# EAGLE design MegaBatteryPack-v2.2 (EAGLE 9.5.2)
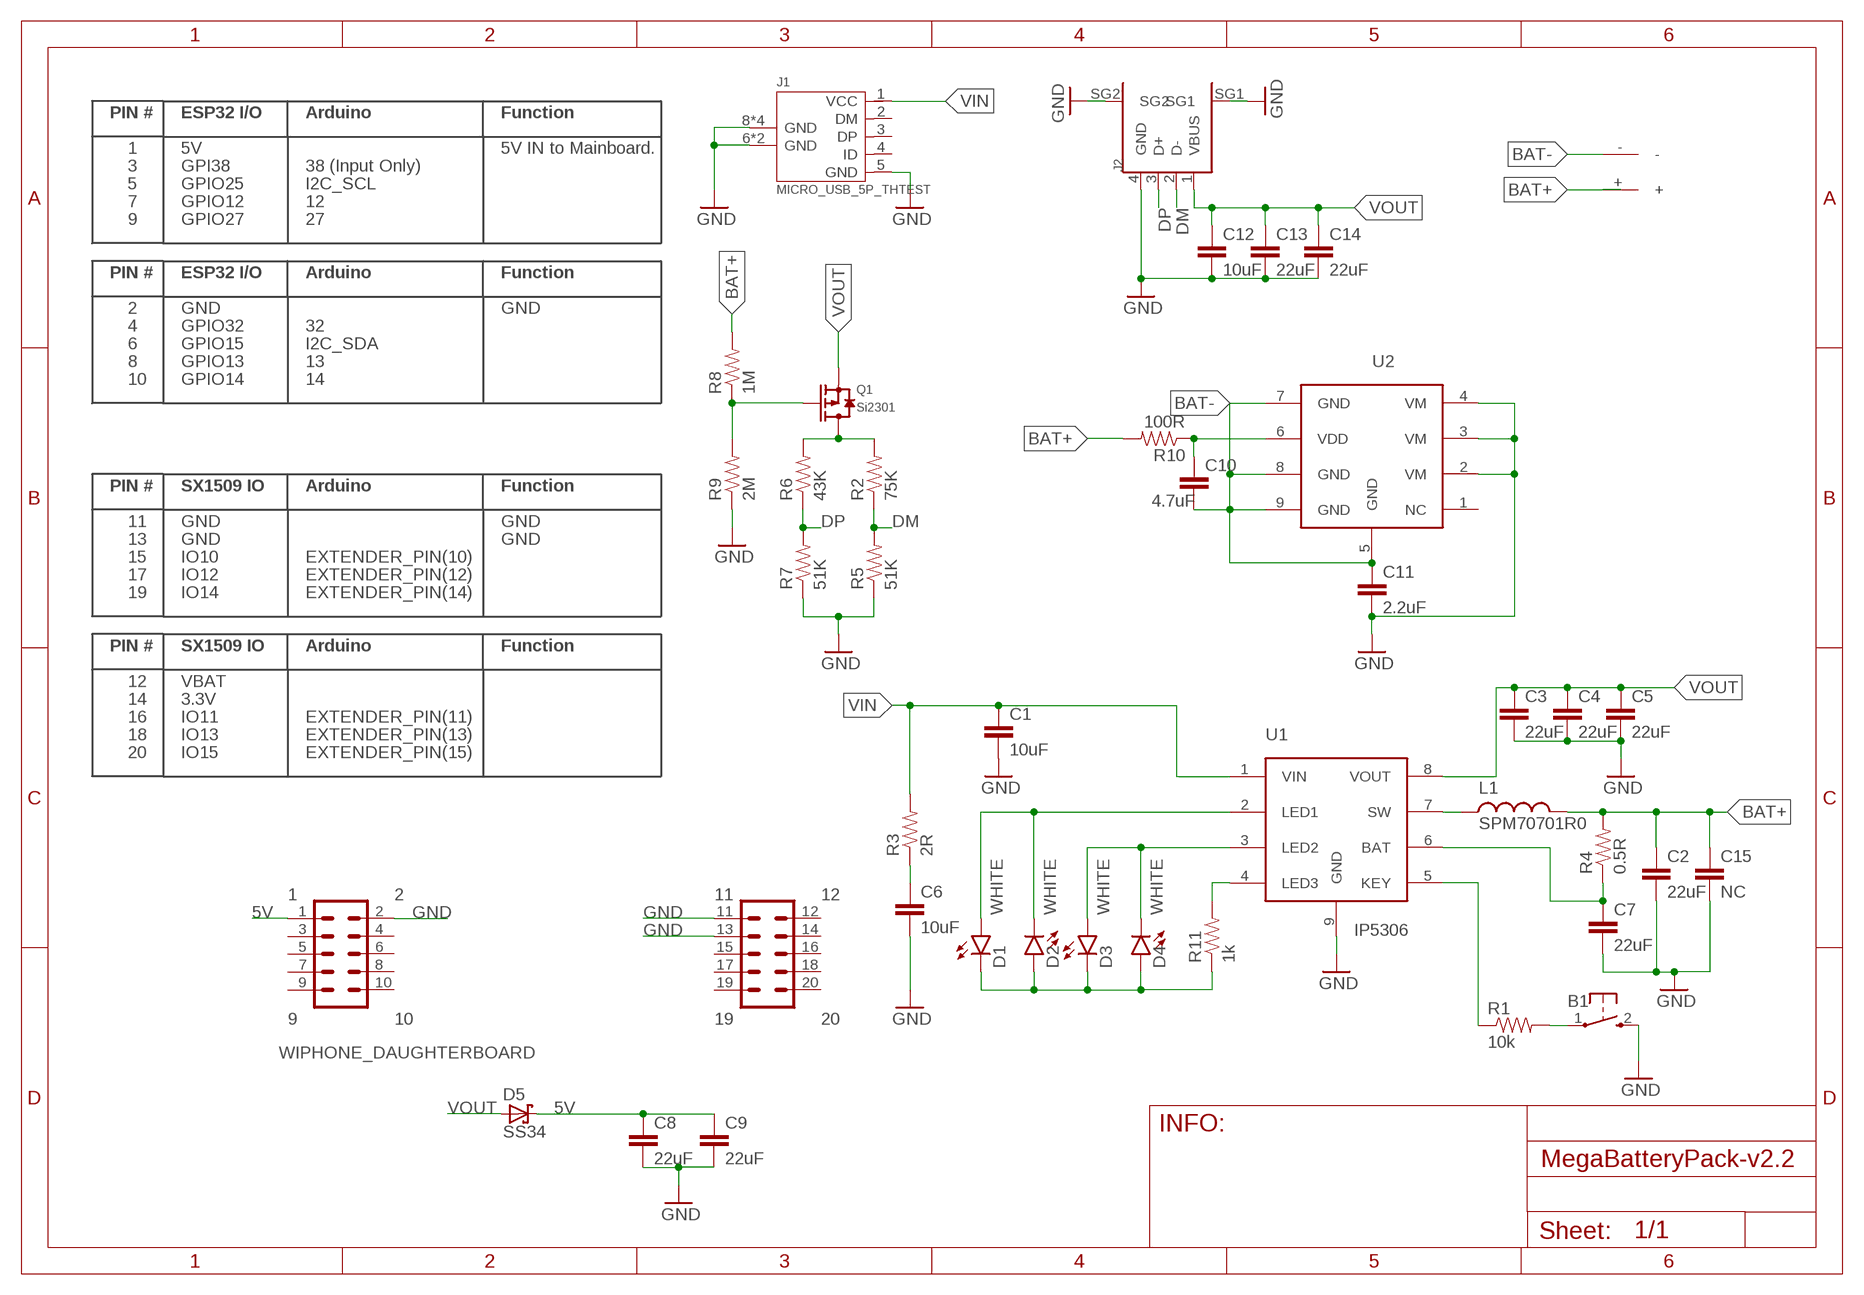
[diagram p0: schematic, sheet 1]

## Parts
B1  BUTTON_3X6X5-90_DEGREE  [3X6X5-90_DEGREE]
C1  10uF  CAP0805  [0805_CAP]
C2  22uF  CAP0805  [0805_CAP]
C3  22uF  CAP0805  [0805_CAP]
C4  22uF  CAP0805  [0805_CAP]
C5  22uF  CAP0805  [0805_CAP]
C6  10uF  CAP0805  [0805_CAP]
C7  22uF  CAP0805  [0805_CAP]
C8  22uF  CAP0805  [0805_CAP]
C9  22uF  CAP0805  [0805_CAP]
C10  4.7uF  CAP  [0603-CAP-L]
C11  2.2uF  CAP0805  [0805_CAP]
C12  10uF  CAP0805  [0805_CAP]
C13  22uF  CAP0805  [0805_CAP]
C14  22uF  CAP0805  [0805_CAP]
C15  NC  CAP0805  [0805_CAP]
D1  WHITE  LED-WHITE0603  [LED-0603]
D2  WHITE  LED-WHITE0603  [LED-0603]
D3  WHITE  LED-WHITE0603  [LED-0603]
D4  WHITE  LED-WHITE0603  [LED-0603]
D5  SS34  DIODE_SCHOTTKEY  [SOD323]
J1  MICRO_USB_5P_THTEST  [B-SMD-5P-WIPHONE-TEST]
J2  USB-A-TYPE-FMAL(4+2P-2.0-90D)  [USB4+2P-2.0-90D]
JP1  WIPHONE_DAUGHTERBOARD  [WIPHONE_DAUGHTERBOARD]
JP904580  JP904580  [JP904580]
L1  SPM70701R0  IND7070  [IND7070]
Q1  Si2301  MOSFET_P  [SOT23-3(SOT95P240X110-3-M)]
R1  10k  RES  [0603-RES-L]
R2  75K  RES  [0603-RES-L]
R3  2R  RES  [0603-RES-L]
R4  0.5R  RES  [0603-RES-L]
R5  51K  RES  [0603-RES-L]
R6  43K  RES  [0603-RES-L]
R7  51K  RES  [0603-RES-L]
R8  1M  RES  [0603-RES-L]
R9  2M  RES  [0603-RES-L]
R10  100R  RES  [0603-RES-L]
R11  1k  RES  [0603-RES-L]
U1  IP5306  [SOP-8(SOP127P600X175-8-M)]
U2  IP3005A  [SOP-8(SOP127P600X175-8-M)]

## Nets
5V: C8.1 C9.1 D5.C JP1.1
BAT+: C2.1 C15.1 JP904580.+ L1.2 R4.2 R8.2 R10.2
BAT-: C10.2 C11.1 JP904580.- U2.5(GND) U2.7(GND) U2.8(GND) U2.9(GND)
DM: J2.2(D-) R2.1 R5.2
DP: J2.3(D+) R6.1 R7.2
GND: B1.2 C1.2 C2.2 C3.2 C4.2 C5.2 C6.2 C7.2 C8.2 C9.2 C11.2 C12.2 C13.2 C14.2 C15.2 J1.5(GND) J1.6(GND) J1.7(GND) J1.8(GND) J1.9(GND) J1.10(GND) J1.11(GND) J2.4(GND) J2.SG1 J2.SG2 JP1.2 JP1.11 JP1.13 R5.1 R7.1 R9.1 U1.9(GND) U2.2(VM) U2.3(VM) U2.4(VM)
N$1: D1.A D2.C U1.2(LED1)
N$2: D1.C D2.A D3.C D4.A R11.1
N$3: D3.A D4.C U1.3(LED2)
N$4: Q1.1(G) R8.1 R9.2
N$5: L1.1 U1.7(SW)
N$6: C6.1 R3.1
N$7: B1.1 R1.2
N$8: R1.1 U1.5(KEY)
N$9: R11.2 U1.4(LED3)
N$10: C7.1 R4.1 U1.6(BAT)
N$13: Q1.3(D) R2.2 R6.2
N$14: C10.1 R10.1 U2.6(VDD)
VIN: C1.1 J1.1(VCC) R3.2 U1.1(VIN)
VOUT: C3.1 C4.1 C5.1 C12.1 C13.1 C14.1 D5.A J2.1(VBUS) Q1.2(S) U1.8(VOUT)
Unconnected: J1.2(DM) J1.3(DP) J1.4(ID) JP1.3 JP1.4 JP1.5 JP1.6 JP1.7 JP1.8 JP1.9 JP1.10 JP1.15 JP1.16 JP1.17 JP1.18 JP1.19 JP1.20 U2.1(NC)

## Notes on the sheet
- 5V IN to Mainboard.
- GND
- GND
- GND

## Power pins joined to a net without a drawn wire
12: JP1.12
14: JP1.14

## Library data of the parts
B1 = WiPhone:BUTTON: Momentary Tactile Switch
C1-C15 = WiPhone:CAP: Capacitor.
D1-D4 = WiPhone:LED-WHITE: White SMD LED
D5 = WiPhone:DIODE_SCHOTTKEY: Schottky barrier diode
J1 = WiPhone:MICRO_USB_5P_TH: MICRO USB B SMD R/A
J2 = WiPhone:USB-A-TYPE-FMAL(4+2P-2.0-90D)
JP1 = WiPhone:WIPHONE_DAUGHTERBOARD
JP904580 = WiPhone:JP904580
L1 = WiPhone:IND: Inductor.
Q1 = WiPhone:MOSFET_P: P-Channel Mosfet
R1-R11 = WiPhone:RES: Resistor.
U1 = WiPhone:IP5306
U2 = WiPhone:IP3005A

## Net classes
1 power: width 0.203 mm

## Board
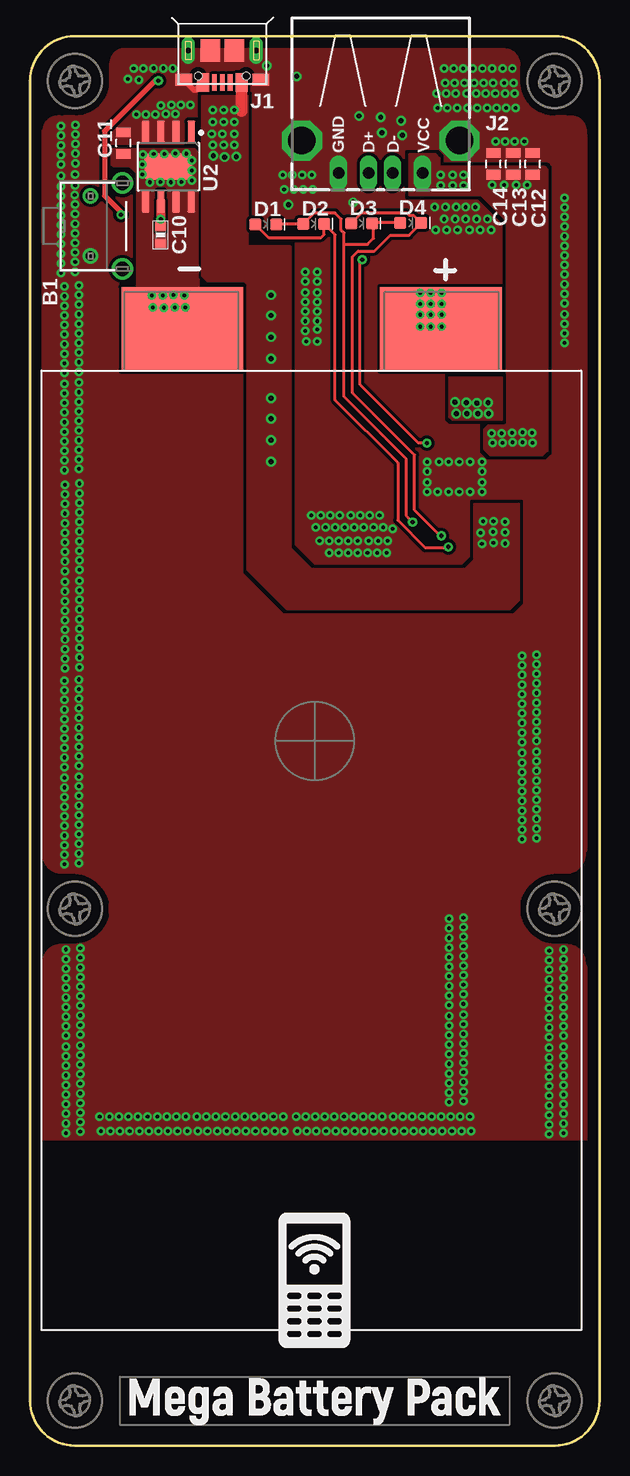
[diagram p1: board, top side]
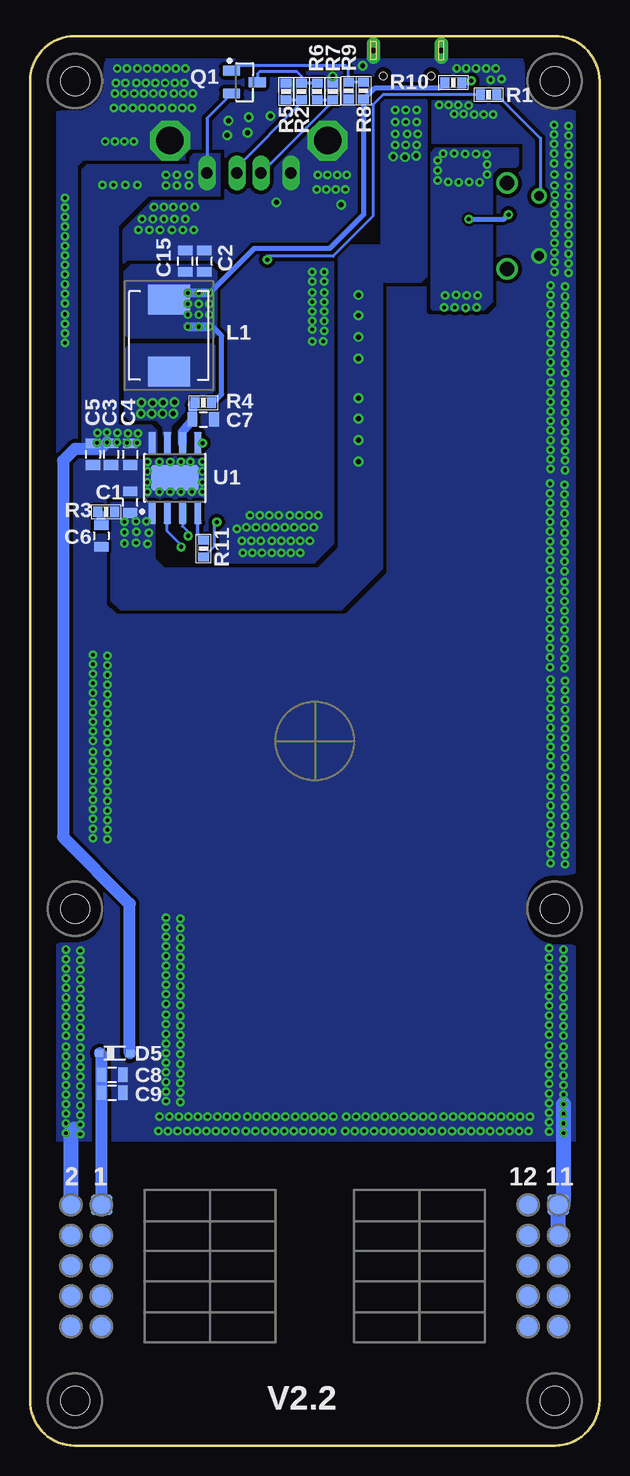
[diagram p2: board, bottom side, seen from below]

Size 47.5 x 117.5 mm. Coordinates in mm from the lower left corner, seen from the top.
Copper layers (1*16): Top 0.035mm / dielectric 1.5mm / Bottom 0.035mm
Design rules "2LDaughterBoards": minimum track width 6mil, minimum drill 0.3mm, track to track 8mil, track to pad 8mil, pad to pad 8mil, via to via 8mil, smd to smd 0mil, copper to edge 16mil, drill to drill 6mil, minimum pad ring 10mil, minimum via ring 8mil, stop-mask expansion 4mil, vias tented up to drill 25mil, thermal gap 10mil

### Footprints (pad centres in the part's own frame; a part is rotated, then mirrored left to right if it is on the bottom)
3X6X5-90_DEGREE = drill 0.8: 1 -2.534,-0.964; 2 2.46,-0.964 | drill 1.2: ANCHOR1 -3.609,1.68; ANCHOR2 3.541,1.68
0805_CAP = smd 0.8 x 1.2: 1 -0.9,0; 2 0.9,0
0603-CAP-L = smd 0.75 x 0.9: 1 -0.7,0; 2 0.7,0
LED-0603 = smd 1 x 1: A -0.877,0; C 0.877,0
SOD323 = smd 0.8 x 0.6: A 1.25,0; C -1.25,0
B-SMD-5P-WIPHONE-TEST = smd 0.98 x 1.52: 1 1.61,-2.383; 5 -1.61,-2.383 | smd 0.406 x 1.372: 2 0.66,-2.383; 3 0,-2.383; 4 -0.66,-2.383 | smd 1.372 x 1.016: 6 -3.2,-2.154; 7 3.2,-2.154 | drill 0.45 pad 1.143 long: 8 2.835,0.284; 9 -2.835,0.284 | smd 1.651 x 1.9: 10 -1,0.284; 11 1,0.284 | hole 0.6: -2,-1.824; 2,-1.824
USB4+2P-2.0-90D = drill 0.95 long: 1 -3.5,2.71; 2 -1,2.71; 3 1,2.71; 4 3.5,2.71 | drill 2.3 octagon: SG1 -6.57,0; SG2 6.57,0
WIPHONE_DAUGHTERBOARD = smd 1.75 x 1.75 bottom: 1 17.78,-38.66; 2 20.32,-38.66; 3 17.78,-41.2; 4 20.32,-41.2; 5 17.78,-43.74; 6 20.32,-43.74; 7 17.78,-46.28; 8 20.32,-46.28; 9 17.78,-48.82; 10 20.32,-48.82; 11 -20.32,-38.66; 12 -17.78,-38.66; 13 -20.32,-41.2; 14 -17.78,-41.2; 15 -20.32,-43.74; 16 -17.78,-43.74; 17 -20.32,-46.28; 18 -17.78,-46.28; 19 -20.32,-48.82; 20 -17.78,-48.82 | hole 2.4: 20,-54.991; -20,-54.991; 20,-13.991; 20,55.009; -20,55.009; -20,-13.991
JP904580 = smd 10.16 x 6.985: + 11.043,44.254; - -10.53,44.254
IND7070 = smd 2.5 x 3.5: 1 -3,0; 2 3,0
SOT23-3(SOT95P240X110-3-M) = smd 1.48 x 0.849: 1 -1.075,0.95; 2 -1.075,-0.95; 3 1.075,0
0603-RES-L = smd 0.75 x 0.9: 1 -0.7,0; 2 0.7,0
SOP-8(SOP127P600X175-8-M) = smd 1.869 x 0.642: 1 -2.893,1.905; 2 -2.893,0.635; 3 -2.893,-0.635; 4 -2.893,-1.905; 5 2.893,-1.905; 6 2.893,-0.635; 7 2.893,0.635; 8 2.893,1.905 | smd 2.2 x 4: 9 0,0

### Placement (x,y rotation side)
B1  6.02,101.64 270 top
C1  39.15,78.64 90 bottom
C2  32.95,98.74 90 bottom
C3  40.75,82.64 270 bottom
C4  39.15,82.64 270 bottom
C5  42.25,82.64 270 bottom
C6  41.55,75.84 270 bottom
C7  33.05,85.54 0 bottom
C8  40.65,30.91 0 bottom
C9  40.65,29.41 0 bottom
C10  10.89,100.92 270 top
C11  7.79,108.58 90 top
C12  41.93,106.85 90 top
C13  40.29,106.85 90 top
C14  38.65,106.85 90 top
C15  34.55,98.74 90 bottom
D1  19.66,101.81 0 top
D2  23.66,101.85 0 top
D3  27.66,101.89 0 top
D4  31.76,101.93 0 top
D5  40.43,32.71 0 bottom
J1  16.04,116.01 0 top
J2  29.25,108.79 180 top
JP1  23.75,58.74 0 top
JP904580  23.24,48.84 0 top
L1  35.91,92.54 90 bottom
Q1  29.61,113.66 0 bottom
R1  9.25,112.61 0 bottom
R2  24.85,112.89 90 bottom
R3  41.15,77.84 0 bottom
R4  33.05,86.94 0 bottom
R5  26.15,112.89 270 bottom
R6  23.55,112.89 90 bottom
R7  22.25,112.89 270 bottom
R8  19.68,112.94 270 bottom
R9  20.92,112.94 90 bottom
R10  12.19,113.62 180 bottom
R11  33.03,74.78 90 bottom
U1  35.41,80.67 90 bottom
U2  11.55,106.62 270 top

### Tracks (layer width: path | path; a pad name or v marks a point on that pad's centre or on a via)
5V
  Bottom 1.016: 41.55,20.1 JP1.1 41.53,29.39 C9.1 C8.1 41.55,32.58 D5.C
BAT+  (via drill 0.3)
  Top 0.762: v34.33,93.28 34.28,93.24 JP904580.+
  Bottom 0.406: R10.2 13.31,113.2 18.72,113.2 R8.2 19.68,102.61 22.51,99.78 28.83,99.78 v32.53,96.08 | R4.2 32.21,86.94 31.51,87.64 31.51,92.52 32.27,93.28 v32.53,93.28
  Bottom 0.762: 35.91,94.86 L1.2 35.37,96.08 v32.53,96.08 | v34.33,93.28 v33.43,93.28 v32.53,93.28
  other vias: 33.43,96.08 34.33,96.08 34.33,95.18 33.43,95.18 32.53,95.18 32.53,94.28 33.43,94.28 34.33,94.28
  pour Bottom (isolate 0.254, no thermals): 32.29,92.34 39.25,92.34 39.61,92.7 39.61,97.88 39.03,98.46 32.57,98.46 31.99,97.88 31.99,92.64
BAT-  (via drill 0.3)
  other vias: 11.21,107.68 9.99,105.32 10.87,105.34 11.75,105.32 12.63,105.34 13.51,106.3 13.51,107.12 13.03,107.7 12.11,107.72 10.31,107.68 9.43,107.62 9.39,106.8 9.39,105.96 13.49,105.46 11.07,95.88 12.89,95.9 11.97,95.92 10.17,95.88 12.07,94.9 10.25,94.88 11.17,94.86 12.97,94.9
  pour Top (rank 2, no thermals): 10.15,94.7 9.61,94.7 8.93,95.38 8.93,106.02 8.47,106.48 8.35,106.6 6.99,106.6 6.79,106.8 6.79,108.1 13.71,108.1 14.07,107.74 14.07,94.84 13.93,94.7 10.17,94.7
  pour Bottom (rank 2, no thermals): 13.93,94.7 9.61,94.7 8.93,95.38 8.93,106.02 8.35,106.6 6.99,106.6 6.79,106.8 6.79,108.1 13.71,108.1 14.07,107.74 14.07,94.84
DM
  Bottom 0.254: R5.2 R2.1 24.85,111.99 30.25,106.59 J2.2
DP
  Bottom 0.254: R6.1 R7.2 22.25,112.08 J2.3
GND  (via drill 0.3, 0.41)
  Top 0.508: J1.5 13.85,113.05 13.85,113 13.69,113 J1.6
  Bottom 1.27: JP1.2 44.07,26.16 43.83,26.4 | JP1.13 JP1.11 2.99,20.52 v2.99,26.86 v2.99,28.46
  other vias: 21.55,103.44 26.95,103.64 37.71,81.2 37.71,82 37.71,80.3 37.71,79.5 33.11,81.2 33.11,82 33.11,80.3 33.11,79.5 34.91,82 34.11,82 35.81,82 36.71,82 34.91,79.5 34.01,79.5 35.81,79.5 36.71,79.5 22.25,114.14 27.45,110.84 29.25,110.74 30.95,110.44 29.35,109.44 31.05,109.24 19.75,115.04 33.75,103.24 34.75,101.34 33.85,101.34 38.45,101.34 37.55,101.34 35.65,101.34 36.65,101.34 35.51,112.72 34.71,112.72 33.91,112.72 12.13,111 11.33,111 35.61,111.52 34.81,111.52 34.01,111.52 38.53,114.8 37.73,114.8 36.93,114.8 36.13,114.8 40.23,114.8 39.43,114.8 38.81,112.72 38.01,112.72 37.21,112.72 36.41,112.72 35.33,114.8 34.53,114.8 40.41,112.72 39.61,112.72 38.63,113.6 37.83,113.6 37.03,113.6 36.23,113.6 40.33,113.6 39.53,113.6 38.91,111.52 38.11,111.52 37.31,111.52 36.51,111.52 35.43,113.6 34.63,113.6 40.51,111.52 39.71,111.52 2.57,104.96 2.57,104.16 2.57,103.36 2.57,102.56 2.59,108.4 2.59,107.6 2.59,106.8 2.57,105.86 21.89,105.92 21.09,105.92 2.59,110 2.59,109.2 23.49,105.92 22.69,105.92 2.57,98.56 2.57,97.76 2.57,101.76 2.57,100.96 2.57,100.16 2.57,99.36 3.77,105.06 3.73,104.26 3.77,103.46 3.77,102.66 3.79,108.5 3.79,107.7 3.79,106.9 3.77,105.96 21.99,104.72 21.19,104.72 3.79,110.1 3.79,109.3 23.59,104.72 22.79,104.72 3.77,98.66 3.77,97.86 3.77,101.86 3.77,101.06 3.77,100.26 3.77,99.46 44.59,95.22 44.59,96.02 44.59,96.82 44.59,97.62 44.59,91.92 44.59,92.72 44.59,93.52 44.59,94.32 44.59,101.62 44.59,102.42 44.59,103.22 44.59,104.02 44.59,98.42 44.59,99.22 44.59,100.02 44.59,100.82 25.85,77.54 25.05,77.54 24.25,77.54 23.45,77.54 29.15,77.54 28.35,77.54 27.55,77.54 26.75,77.54 26.25,76.54 25.45,76.54 24.65,76.54 23.85,76.54 29.45,76.54 28.65,76.54 27.85,76.54 27.05,76.54 27.35,75.44 26.55,75.44 25.75,75.44 24.95,75.44 30.25,76.44 29.85,75.44 29.05,75.44 28.25,75.44 27.35,74.44 26.55,74.44 25.75,74.44 24.95,74.44 24.15,75.44 29.75,74.44 28.95,74.44 28.15,74.44 10.47,110.98 9.67,110.98 8.87,110.98 10.93,111.72 13.39,111.76 12.59,111.76 11.79,111.76 11.91,114.82 11.11,114.82 10.31,114.82 9.45,114.8 8.65,114.8 9.07,113.86 8.17,113.92 29.39,27.42 28.59,27.42 27.79,27.42 26.99,27.42 32.69,27.42 31.89,27.42 31.09,27.42 30.29,27.42 35.89,27.42 35.09,27.42 34.29,27.42 33.49,27.42 36.69,27.42 22.99,27.42 22.19,27.42 26.19,27.42 25.39,27.42 24.59,27.42 23.79,27.42 29.49,26.22 28.69,26.22 27.89,26.22 27.09,26.22 32.79,26.22 31.99,26.22 31.19,26.22 30.39,26.22 35.99,26.22 35.19,26.22 34.39,26.22 33.59,26.22 36.79,26.22 23.09,26.22 22.29,26.22 26.29,26.22 25.49,26.22 24.69,26.22 23.89,26.22 43.31,33.16 43.31,32.36 43.31,31.56 43.31,30.76 43.31,36.46 43.31,35.66 43.31,34.86 43.31,34.06 43.31,39.66 43.31,38.86 43.31,38.06 43.31,37.26 43.31,41.26 43.31,40.46 43.31,26.76 43.31,25.96 43.31,29.96 43.31,29.16 43.31,28.36 43.31,27.56 44.51,33.26 44.51,32.46 44.51,31.66 44.51,30.86 44.51,36.56 44.51,35.76 44.51,34.96 44.51,34.16 44.51,39.76 44.51,38.96 44.51,38.16 44.51,37.36 44.51,41.36 44.51,40.56 44.51,26.86 44.51,26.06 44.51,30.06 44.51,29.26 44.51,28.46 44.51,27.66 13.01,27.42 12.21,27.42 11.41,27.42 10.61,27.42 16.31,27.42 15.51,27.42 14.71,27.42 13.91,27.42 19.51,27.42 18.71,27.42 17.91,27.42 17.11,27.42 21.11,27.42 20.31,27.42 6.61,27.42 5.81,27.42 9.81,27.42 9.01,27.42 8.21,27.42 7.41,27.42 13.11,26.22 12.31,26.22 11.51,26.22 10.71,26.22 16.41,26.22 15.61,26.22 14.81,26.22 14.01,26.22 19.61,26.22 18.81,26.22 18.01,26.22 17.21,26.22 21.21,26.22 20.41,26.22 6.71,26.22 5.91,26.22 9.91,26.22 9.11,26.22 8.31,26.22 7.51,26.22 2.99,33.26 2.99,32.46 2.99,31.66 2.99,30.86 2.99,36.56 2.99,35.76 2.99,34.96 2.99,34.16 2.99,39.76 2.99,38.96 2.99,38.16 2.99,37.36 2.99,41.36 2.99,40.56 2.99,26.06 2.99,30.06 2.99,29.26 2.99,27.66 4.19,33.36 4.19,32.56 4.19,31.76 4.19,30.96 4.19,36.66 4.19,35.86 4.19,35.06 4.19,34.26 4.19,39.86 4.19,39.06 4.19,38.26 4.19,37.46 4.19,41.46 4.19,40.66 4.19,26.96 4.19,26.16 4.19,30.16 4.19,29.36 4.19,28.56 4.19,27.76 2.87,55.66 2.87,54.86 2.87,54.06 2.87,53.26 2.87,58.96 2.87,58.16 2.87,57.36 2.87,56.56 2.87,62.16 2.87,61.36 2.87,60.56 2.87,59.76 2.87,63.76 2.87,62.96 2.87,49.26 2.87,48.46 2.87,52.46 2.87,51.66 2.87,50.86 2.87,50.06 4.07,55.76 4.07,54.96 4.07,54.16 4.07,53.36 4.07,59.06 4.07,58.26 4.07,57.46 4.07,56.66 4.07,62.26 4.07,61.46 4.07,60.66 4.07,59.86 4.07,63.86 4.07,63.06 4.07,49.36 4.07,48.56 4.07,52.56 4.07,51.76 4.07,50.96 4.07,50.16 2.91,72 2.91,71.2 2.91,70.4 2.91,69.6 2.91,75.3 2.91,74.5 2.91,73.7 2.91,72.9 2.91,78.5 2.91,77.7 2.91,76.9 2.91,76.1 2.91,80.1 2.91,79.3 2.91,65.6 2.91,64.8 2.91,68.8 2.91,68 2.91,67.2 2.91,66.4 4.11,72.1 4.11,71.3 4.11,70.5 4.11,69.7 4.11,75.4 4.11,74.6 4.11,73.8 4.11,73 4.11,78.6 4.11,77.8 4.11,77 4.11,76.2 4.11,80.2 4.11,79.4 4.11,65.7 4.11,64.9 4.11,68.9 4.11,68.1 4.11,67.3 4.11,66.5 2.87,88.52 2.87,87.72 2.87,86.92 2.87,86.12 2.87,91.82 2.87,91.02 2.87,90.22 2.87,89.42 2.87,95.02 2.87,94.22 2.87,93.42 2.87,92.62 2.87,96.62 2.87,95.82 2.87,82.12 2.87,81.32 2.87,85.32 2.87,84.52 2.87,83.72 2.87,82.92 4.07,88.62 4.07,87.82 4.07,87.02 4.07,86.22 4.07,91.92 4.07,91.12 4.07,90.32 4.07,89.52 4.07,95.12 4.07,94.32 4.07,93.52 4.07,92.72 4.07,96.72 4.07,95.92 4.07,82.22 4.07,81.42 4.07,85.42 4.07,84.62 4.07,83.82 4.07,83.02 34.95,35.82 34.95,35.02 34.95,34.22 34.95,33.42 34.95,39.12 34.95,38.32 34.95,37.52 34.95,36.72 34.95,42.32 34.95,41.52 34.95,40.72 34.95,39.92 34.95,43.92 34.95,43.12 34.95,29.42 34.95,28.62 34.95,32.62 34.95,31.82 34.95,31.02 34.95,30.22 36.15,35.92 36.15,35.12 36.15,34.32 36.15,33.52 36.15,39.22 36.15,38.42 36.15,37.62 36.15,36.82 36.15,42.42 36.15,41.62 36.15,40.82 36.15,40.02 36.15,44.02 36.15,43.22 36.15,29.52 36.15,28.72 36.15,32.72 36.15,31.92 36.15,31.12 36.15,30.32 41.05,57.74 41.05,56.94 41.05,56.14 41.05,55.34 41.05,61.04 41.05,60.24 41.05,59.44 41.05,58.64 41.05,64.24 41.05,63.44 41.05,62.64 41.05,61.84 41.05,65.84 41.05,65.04 41.05,51.34 41.05,50.54 41.05,54.54 41.05,53.74 41.05,52.94 41.05,52.14 42.25,57.84 42.25,57.04 42.25,56.24 42.25,55.44 42.25,61.14 42.25,60.34 42.25,59.54 42.25,58.74 42.25,64.34 42.25,63.54 42.25,62.74 42.25,61.94 42.25,65.94 42.25,65.14 42.25,51.44 42.25,50.64 42.25,54.64 42.25,53.84 42.25,53.04 42.25,52.24 34.55,102.24 35.45,102.24 37.15,103.24 34.65,103.24 35.55,103.24 36.35,103.24 36.35,102.24 37.25,102.24 38.15,102.24 40.43,108.72 39.63,108.72 38.83,108.72 41.23,108.72 22.95,96.14 22.95,95.34 22.95,94.54 22.95,93.74 23.95,93.04 22.95,92.94 22.95,97.84 22.95,97.04 23.95,96.14 23.95,95.34 23.95,94.54 23.95,93.74 23.05,92.04 23.95,92.04 23.95,97.84 23.95,97.04
  pour Top (isolate 0.254, rank 5, no thermals): -0.22,117.52 -0.22,25.55 47.8,25.55 47.8,117.52
  pour Bottom (isolate 0.305, rank 5, no thermals): -0.09,117.47 -0.09,25.5 47.93,25.5 47.93,117.47
N$1  (via drill 0.35)
  Top 0.254: v34.89,74.92 34.81,74.84 32.97,74.84 30.67,77.14 30.67,81.94 25.45,87.16 25.45,100.93 D2.C 24.53,100.96 24.27,100.7 19.89,100.7 D1.A
  Bottom 0.254: v34.89,74.92 34.89,75.08 36.05,76.24 U1.2
N$2  (via drill 0.35)
  Top 0.254: D4.A 28.65,101.93 | 28.65,101.93 28.57,101.93 D3.C | D1.C 22.74,101.81 D2.A 23.67,102.74 25.45,102.74 25.95,102.24 25.95,101.34 26.19,101.1 26.19,100.14 | 26.19,100.14 28.15,100.14 28.65,100.64 28.65,101.93 | v31.92,76.99 31.37,77.54 31.37,82.26 26.19,87.44 26.19,100.14
  Bottom 0.254: R11.1 32.15,74.96 32.15,76.76 v31.92,76.99
N$3  (via drill 0.35)
  Top 0.254: D3.A 27.65,102.76 31.43,102.76 31.65,102.54 32.02,102.54 D4.C 31.61,100.9 30.05,100.9 28.73,99.58 27.37,99.58 26.91,99.12 26.91,87.74 32.07,82.58 32.07,77.98 32.9,77.15 34.21,75.84 v34.31,75.84
  Bottom 0.254: U1.3 34.78,76.65 34.31,76.18 v34.31,75.84
N$4
  Bottom 0.254: R8.1 R9.2 20.92,114.81 21.16,115.05 30.25,115.05 Q1.1
N$5  (via drill 0.41)
  other vias: 38.25,86.04 35.55,86.04 36.45,86.04 37.35,86.04 38.21,86.94 35.45,86.98 36.39,86.94 37.27,86.92
  pour Bottom (isolate 0.254, no thermals): 35.75,84.24 35.75,85.02 34.13,86.64 34.13,87.5 32.55,87.5 32.05,88 32.05,91.66 32.17,91.76 34.13,91.76 39.17,91.78 39.61,91.34 39.61,85.92 39.21,85.52 36.99,85.52 36.39,84.92 36.39,84.24
  pour Top (isolate 0.254, no thermals): 35.21,85.5 34.97,85.74 34.97,89.06 39.37,89.06 39.37,85.5
N$6
  Bottom 0.762: C6.1 41.55,77.54 R3.1
N$7
  Bottom 0.254: R1.2 4.93,108.99 4.93,104.29 B1.1
N$8  (via drill 0.35)
  Top 0.254: v33.11,83.58 32.39,83.58 27.51,88.46 27.51,98.67 v27.71,98.87
  Bottom 0.254: R1.1 18.08,112.61 18.9,111.79 18.9,102.47 22.22,99.15 27.77,99.15 27.71,99.09 v27.71,98.87 | U1.5 33.49,83.58 v33.11,83.58
N$9
  Bottom 0.305: U1.4 33.51,75.96 R11.2
N$10
  Bottom 0.762: R4.1 33.95,86.74 C7.1 34.78,84.51 U1.6
N$13
  Bottom 0.254: R6.2 R2.2 24.85,114.14 25.25,114.54 28.35,114.54 28.53,114.36 Q1.3
N$14  (via drill 0.35)
  Top 0.406: v10.71,113.78 10.43,113.78 6.23,109.58 6.23,104.18 7.59,102.82 v7.59,102.62
  Top 0.762: U2.6 v10.91,102.25 v10.91,102.24 10.91,101.64 C10.1
  Bottom 0.406: R10.1 10.87,113.62 v10.71,113.78 | v10.91,102.24 7.97,102.24 v7.59,102.62
VIN  (via drill 0.3, 0.41)
  Top 0.965: J1.1 17.65,111.24
  other vias: 16.23,107.42 17.21,107.46 15.29,107.52 20.11,95.92 20.11,94.22 20.11,92.42 20.11,90.62 20.11,87.32 20.11,85.62 20.11,83.82 20.11,82.02 38.63,76.16 39.63,76.12 38.65,75.26 37.57,76.1 39.63,75.2 38.65,77.06 39.63,77.02 37.69,75.18 37.79,77.04 15.25,111.34 16.15,111.34 17.05,111.34 17.05,110.34 16.15,110.34 15.25,110.34 17.05,109.34 16.05,109.34 15.15,109.34 15.25,108.44 16.15,108.44 17.05,108.44
  pour Top (isolate 0.254, no thermals): 37.07,78.54 40.76,78.54 40.76,70.45 40.01,69.7 21.43,69.7 18.15,72.98 18.15,96.8 17.91,97.04 14.83,97.04 14.37,97.5 14.37,112.54 18.15,112.54 18.15,100.1 18.23,100.02 21.67,100.02 21.73,99.96 21.73,74.82 23.44,73.11 36.32,73.11 37.07,73.86
  pour Bottom (isolate 0.254, no thermals): 37.07,78.56 40.71,78.56 40.71,70.46 39.97,69.72 21.49,69.72 18.11,73.1 18.11,97.04 14.87,97.04 14.41,97.5 14.41,112.06 14.65,112.3 18.03,112.3 18.21,112.12 18.21,100.12 18.29,100.04 21.73,100.04 21.79,99.98 21.79,74.84 23.5,73.13 36.32,73.13 37.07,73.88
VOUT  (via drill 0.3)
  Bottom 0.254: Q1.2 32.75,110.65 J2.1
  Bottom 1.016: v41.07,83.64 41.61,83.1 43.75,83.1 44.75,82.1 44.75,50.74 39.18,45.17 D5.A
  other vias: 38.51,84.4 38.57,83.58 39.33,84.4 39.41,83.6 41.93,83.6 40.21,84.44 34.25,105.94 34.25,105.04 35.25,105.94 36.15,105.94 35.25,105.04 36.15,105.04 41.45,105.08 40.55,105.08 39.55,105.08 38.55,105.08 40.25,83.64 41.07,84.46 41.89,84.44
  pour Bottom (isolate 0.254, rank 2, no thermals): 42.85,82.64 37.03,82.64 36.93,82.74 36.93,84.6 37.33,85 39.95,85 39.97,85.02 40.13,85.02 40.13,101.7 37.61,104.22 31.65,104.22 31.65,107.64 33.85,107.64 34.15,107.34 34.15,106.74 42.75,106.74 43.15,106.34 43.15,82.94
  pour Top (isolate 0.254, rank 3, no thermals): 38.25,85.08 39.61,85.08 39.77,85.24 39.77,102.06 37.63,104.2 31.65,104.2 31.65,107.68 33.81,107.68 34.15,107.34 34.15,106.64 42.89,106.64 43.15,106.38 43.15,82.94 42.75,82.54 38.39,82.54 37.91,83.02 37.91,84.74

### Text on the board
bPlace: V2.2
